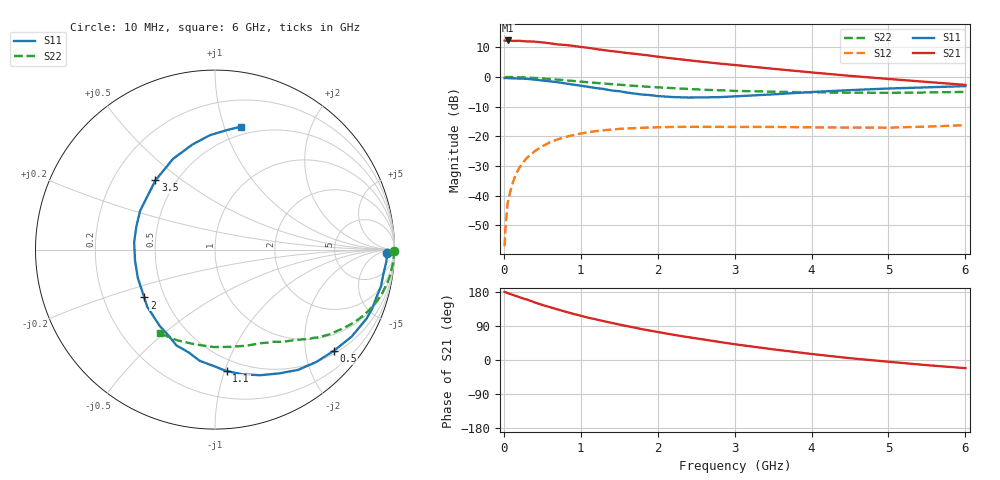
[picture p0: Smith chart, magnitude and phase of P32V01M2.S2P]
! SIEMENS Small Signal Semiconductors
! BFP181
! Si NPN RF Bipolar Junction Transistor in SOT143
! VCE = 2 V  IC = 1.2 mA
! Common Emitter S-Parameters:  March  1996
# GHz  S  MA  R  50
!  f  S11  S21  S12  S22
! GHz  MAG  ANG  MAG  ANG  MAG  ANG  MAG  ANG
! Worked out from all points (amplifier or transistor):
!   36 points, 10 MHz to 6 GHz, reference 50 ohm
!   highest |S21| = 12.3 dB at 50 MHz (marker M1)
!   |S21| within 3 dB of that: start of sweep to 1.229 GHz
!   unconditionally stable (mu >= 1): 2.862 GHz to end of sweep
!   at 250 MHz: K = 0.08, MSG = 20.5 dB, |S12| = -28.8 dB
!   at 1.4 GHz: K = 0.53, MSG = 13.2 dB, |S12| = -17.7 dB
!   at 6 GHz: K = 1.26, MAG = 3.7 dB, |S12| = -16.3 dB
!   S11 on the Smith chart (normalised r, x): 10 MHz: 40, -17; 500 MHz: 0.56, -2.60; 1.1 GHz: 0.40, -1.02; 2 GHz: 0.38, -0.26; 3.5 GHz: 0.39, +0.40; 6 GHz: 0.42, +1.14
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0.01  0.9584 -1.0  4.098 179.6  0.0014 88.8  0.9982 -0.3
0.02  0.9595 -1.6  4.085 179.2  0.0027 88.9  0.9914 -0.7
0.05  0.9568 -4.1  4.124 176.5  0.0076 89.4  0.9959 -1.9
0.1  0.9478 -8.5  4.071 173.0  0.0142 83.3  0.9961 -3.8
0.2  0.9379 -16.5  4.082 165.9  0.0292 79.9  0.9878 -7.6
0.4  0.9026 -32.5  3.941 152.1  0.0559 69.5  0.9621 -14.8
0.5  0.8694 -40.5  3.823 145.3  0.0675 64.0  0.9431 -18.2
0.6  0.8432 -47.9  3.696 139.4  0.0794 59.4  0.923 -21.4
0.8  0.7773 -62.5  3.46 127.6  0.0971 51.0  0.8799 -27.0
0.9  0.7439 -70.2  3.346 121.9  0.1043 47.2  0.8563 -29.6
1.1  0.6804 -84.5  3.099 111.5  0.1169 40.4  0.8124 -34.2
1.3  0.6258 -97.7  2.833 102.5  0.1263 34.4  0.7745 -38.3
1.5  0.5751 -112.0  2.646 93.6  0.1329 29.4  0.7389 -41.6
1.8  0.5046 -133.2  2.373 81.1  0.139 23.4  0.6929 -46.3
2  0.476 -145.9  2.195 73.9  0.1416 19.8  0.6678 -49.1
2.2  0.458 -160.0  2.046 66.7  0.1435 16.6  0.6477 -52.1
2.8  0.4567 163.7  1.682 47.7  0.144 9.7  0.5956 -60.5
3.5  0.5088 130.7  1.373 28.2  0.1436 4.8  0.5644 -71.3
4  0.5572 114.8  1.192 15.9  0.1413 2.6  0.5494 -80.5
4.5  0.5994 102.0  1.044 4.8  0.14 1.5  0.543 -90.8
5.5  0.6675 84.7  0.824 -13.6  0.1454 3.5  0.5473 -112.3
6  0.7009 78.0  0.735 -21.5  0.1537 3.3  0.5589 -123.4
